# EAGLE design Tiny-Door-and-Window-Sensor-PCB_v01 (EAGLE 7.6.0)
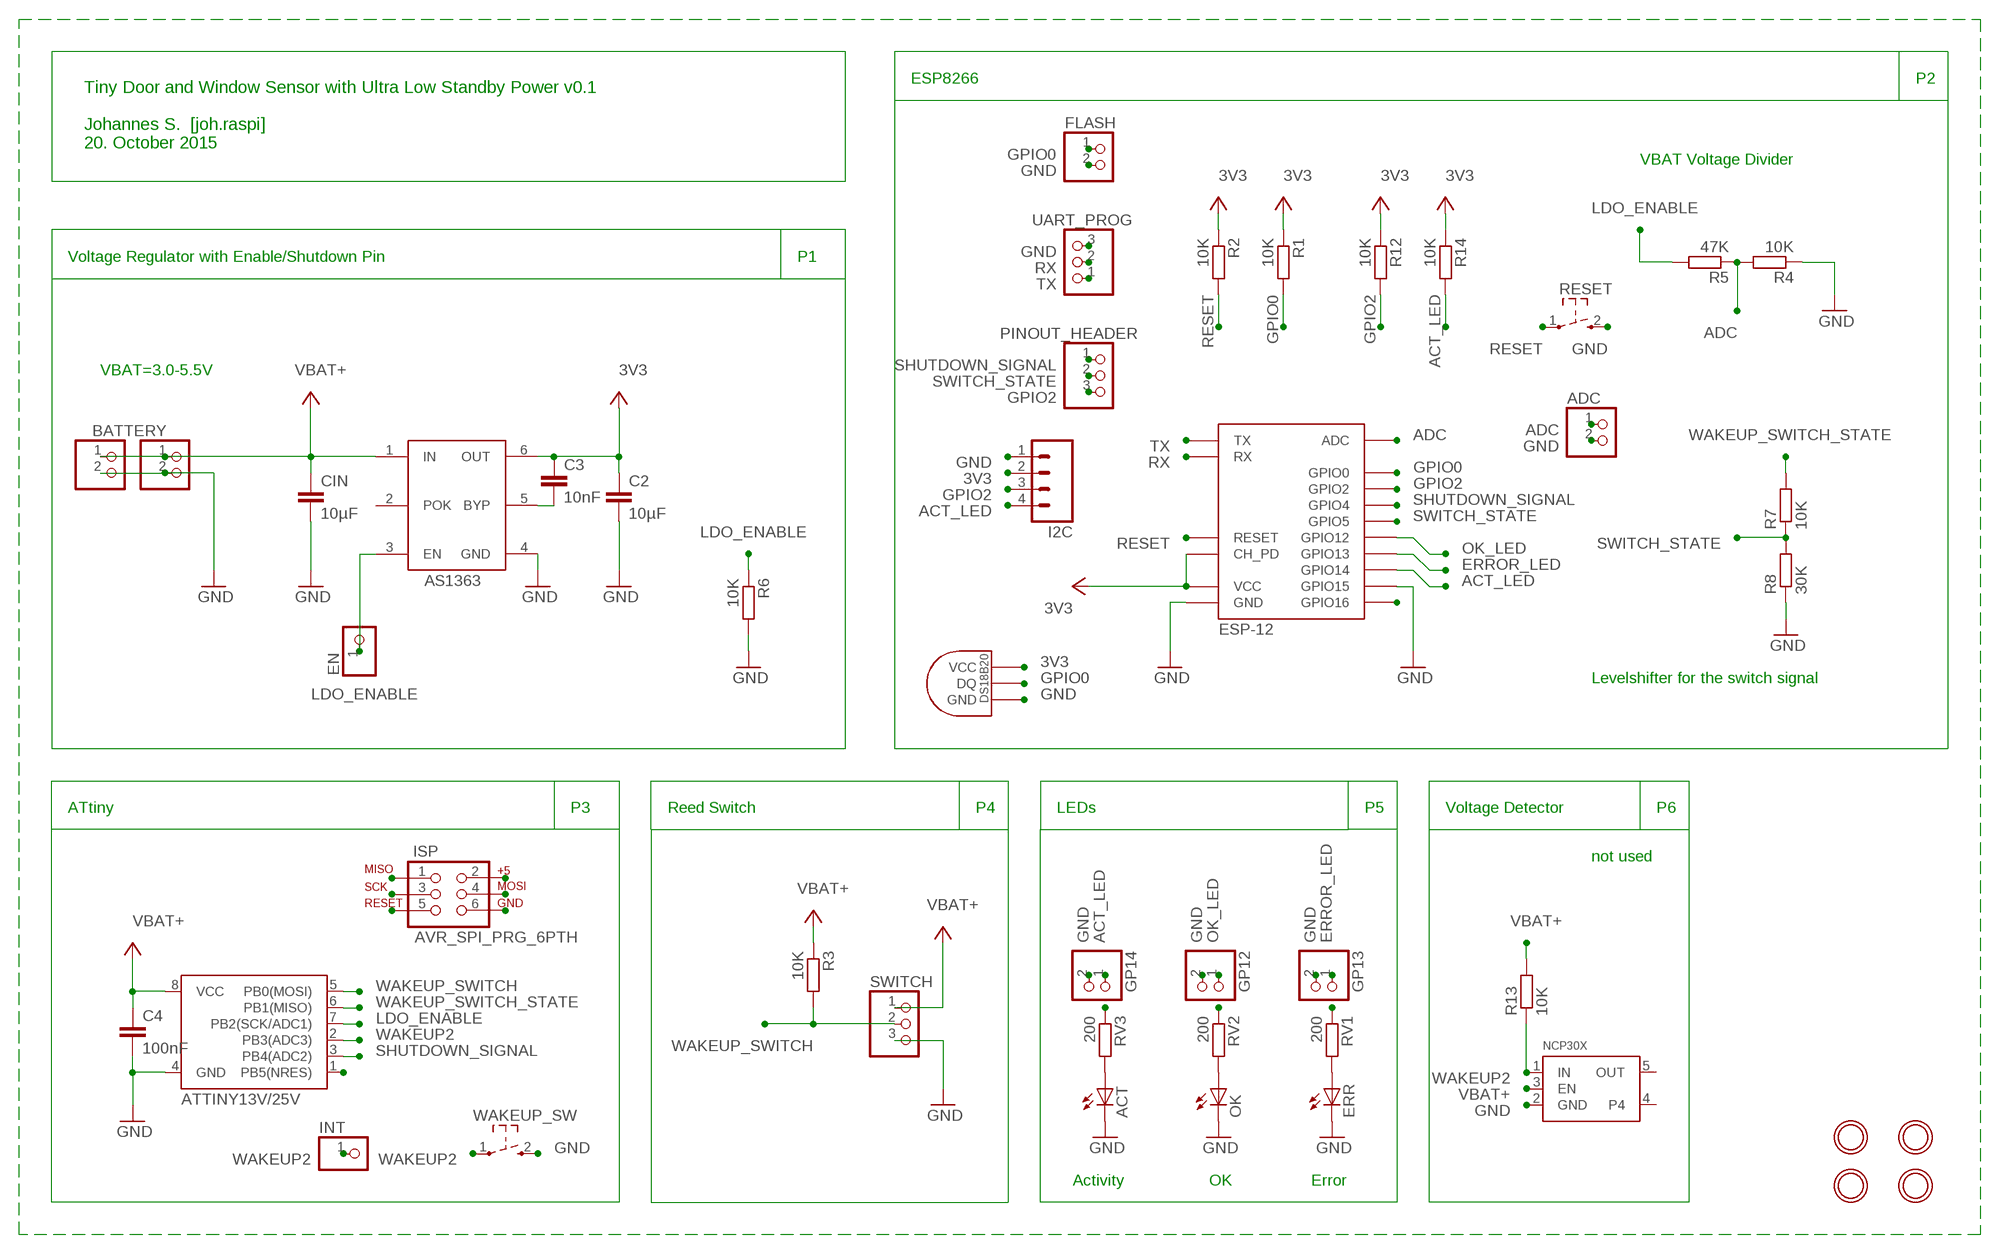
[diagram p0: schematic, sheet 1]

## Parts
ACT  LEDSML0805  [SML0805]
ADC  HEADER-1X2ROUND  [1X02_ROUND]
BATTERY  HEADER-1X2  [1X02_OVAL]
C2  10µF  C-EUC0805  [C0805]
C3  10nF  C-EUC0805  [C0805]
C4  100nF  C-EUC0805  [C0805]
CHARGE  HEADER-1X2  [1X02_OVAL]
CIN  10µF  C-EUC0805  [C0805]
EN  PINHD-1X1  [1X01]
ERR  LEDSML0805  [SML0805]
FLASH  HEADER-1X2ROUND  [1X02_ROUND]
GP12  HEADER-1X2ROUND  [1X02_ROUND]
GP13  HEADER-1X2ROUND  [1X02_ROUND]
GP14  HEADER-1X2ROUND  [1X02_ROUND]
I2C  M04PTH  [1X04]
IC1  AS1363  [SOT23-6]
INT  PINHD-1X1  [1X01]
ISP  AVR_SPI_PRG_6PTH  [2X3]
NCP30X  VREG_SOT23-5  [SOT23-5]
OK  LEDSML0805  [SML0805]
PINOUT_HEADER  PINHD-1X3  [1X03]
R1  10K  R-EU_R0805  [R0805]
R2  10K  R-EU_R0805  [R0805]
R3  10K  R-EU_R0805  [R0805]
R4  10K  R-EU_R0805  [R0805]
R5  47K  R-EU_R0805  [R0805]
R6  10K  R-EU_R0805  [R0805]
R7  10K  R-EU_R0805  [R0805]
R8  30K  R-EU_R0805  [R0805]
R12  10K  R-EU_R0805  [R0805]
R13  10K  R-EU_R0805  [R0805]
R14  10K  R-EU_R0805  [R0805]
RESET  SW_TACT_2P-3X6  [SW_TACT_3X6]
RV1  200  R-EU_R0805  [R0805]
RV2  200  R-EU_R0805  [R0805]
RV3  200  R-EU_R0805  [R0805]
SWITCH  PINHD-1X3  [1X03]
U$1  DS1820TO92  [DS1820]
U$2  ATTINY13V/25V  ATTINY13SOIC  [SO08]
U$3  ESP-12  [ESP-12]
U$4  MOUNTINGHOLE2.5_THICK  [MOUNTINGHOLE_2.5_PLATED_THICK]
U$5  MOUNTINGHOLE2.5_THICK  [MOUNTINGHOLE_2.5_PLATED_THICK]
U$6  MOUNTINGHOLE2.5_THICK  [MOUNTINGHOLE_2.5_PLATED_THICK]
U$7  MOUNTINGHOLE2.5_THICK  [MOUNTINGHOLE_2.5_PLATED_THICK]
UART_PROG  PINHD-1X3  [1X03]
WAKEUP_SW  SW_TACT_2P-3X6  [SW_TACT_3X6]

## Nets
3V3: C2.1 C3.1 I2C.2 IC1.6(OUT) R1.1 R2.1 R12.1 R14.1 U$1.VDD(VCC) U$3.CH_PD U$3.VCC ; supply symbol labelled VCC
ACT_LED: GP14.1 I2C.4 R14.2 RV3.1 U$3.GPIO14
ADC: ADC.1 R4.2 R5.1 U$3.ADC
AT_RESET: ISP.5 U$2.1(PB5(NRES))
ERROR_LED: GP13.1 RV1.1 U$3.GPIO13
GND: ACT.C ADC.2 BATTERY.2 C2.2 C4.2 CHARGE.2 CIN.2 ERR.C FLASH.2 GP12.2 GP13.2 GP14.2 I2C.1 IC1.4(GND) ISP.6 NCP30X.2(GND) OK.C R4.1 R6.2 R8.1 RESET.2 SWITCH.3 U$1.GND U$2.4(GND) U$3.GND U$3.GPIO15 UART_PROG.3 WAKEUP_SW.2
GPIO0: FLASH.1 R1.2 U$1.DQ U$3.GPIO0
GPIO2: I2C.3 PINOUT_HEADER.3 R12.2 U$3.GPIO2
LDO_ENABLE: EN.1 IC1.3(EN) ISP.3 R5.2 R6.1 U$2.7(PB2(SCK/ADC1))
N$4: C3.2 IC1.5(BYP)
N$8: ACT.A RV3.2
N$10: OK.A RV2.2
N$11: ERR.A RV1.2
N$15: U$3.GPIO16
OK_LED: GP12.1 RV2.1 U$3.GPIO12
RESET: R2.2 RESET.1 U$3.RESET
RX: U$3.RX UART_PROG.2
SHUTDOWN_SIGNAL: PINOUT_HEADER.1 U$2.3(PB4(ADC2)) U$3.GPIO4
SWITCH_STATE: PINOUT_HEADER.2 R7.1 R8.2 U$3.GPIO5
TX: U$3.TX UART_PROG.1
VBAT+: BATTERY.1 C4.1 CHARGE.1 CIN.1 IC1.1(IN) ISP.2 NCP30X.3(EN) R3.1 R13.2 SWITCH.1 U$2.8(VCC) ; supply symbol labelled VCC
WAKEUP2: INT.1 NCP30X.1(IN) R13.1 U$2.2(PB3(ADC3)) WAKEUP_SW.1
WAKEUP_SWITCH: ISP.4 R3.2 SWITCH.2 U$2.5(PB0(MOSI))
WAKEUP_SWITCH_STATE: ISP.1 R7.2 U$2.6(PB1(MISO))
Unconnected: IC1.2(POK) NCP30X.4 NCP30X.5(OUT)

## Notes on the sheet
- ESP8266 | P2
- Tiny Door and Window Sensor with Ultra Low Standby Power v0.1
  
  Johannes S.  [joh.raspi]
  20. October 2015
- VBAT Voltage Divider
- Voltage Regulator with Enable/Shutdown Pin | P1
- VBAT=3.0-5.5V
- Levelshifter for the switch signal
- ATtiny | P3 | Reed Switch | P4 | LEDs | P5 | Voltage Detector | P6
- not used
- Activity | OK | Error

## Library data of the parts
ACT ERR OK = led:LED: LED
ADC BATTERY CHARGE FLASH GP12-GP14 = microbuilder:HEADER-1X2: PIN HEADER
C2-C4 CIN = resistor:C-EU: CAPACITOR, European symbol
EN INT = pinhead:PINHD-1X1: PIN HEADER
I2C = SparkFun:M04: Header 4 Standard 4-pin 0.1" header. Use with straight break away headers (SKU : PRT-00116), right angle break away headers (PRT-00553), swiss pins (PRT-00743), machine pins (PRT-00117), and female headers (PRT-00115). Molex polarized connector foot print use with SKU : PRT-08231 with associated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
IC1 = joh_as1363:AS1363: 500mA ultra-low-dropout linear regulator 1.2V-5V 40µA quiescen current Source: http://ams.com/eng/content/download/12507/219217/12422
ISP = SparkFun:AVR_SPI_PRG_6: AVR ISP 6 Pin This is the reduced ISP connector for AVR programming. Common on Arduino. This footprint will take up less PCB space and can be used with a 10-pin to 6-pin adapter such as SKU: BOB-08508
NCP30X = microbuilder:VREG_SOT23-5: SOT23-5 Fixed Voltage Regulators To better organise some of the SOT23-5 fixed voltage regulators in this library, this new part was created. Part Current Out V Out V In V Dropout Digikey Part No. ADP121 150mA 3.3V 3.4-5.5V 0.09V @ 150mA ADP121-AUJZ33R7CT-ND ADP121 150mA 3.0V 3.1-5.5V 0.09V @ 150mA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
PINOUT_HEADER SWITCH UART_PROG = pinhead:PINHD-1X3: PIN HEADER
R1-R8 R12-R14 RV1-RV3 = resistor:R-EU_: RESISTOR, European symbol
RESET WAKEUP_SW = dp-devices:SW_TACT_2P
U$1 = Ava:DS1820: DS18B20 Programmable Resolution 1-Wire Digital Thermometer Description The DS18B20 digital thermometer provides 9-bit to 12-bit Celsius temperature measurements and has an alarm function with nonvolatile user-programmable upper and lower trigger points. The DS18B20 communicates over a 1-Wire® bus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
U$2 = SparkFun:ATTINY13
U$3 = johs_esp8266_lib_frank_esp12e_mod:ESP-12: ESP8266 Wifi Module ESP-12; DIMENSIONS: 24.0 x 16.0 mm; PINS: 16; PITCH: 0.078" / 2 mm
U$4-U$7 = microbuilder:MOUNTINGHOLE: Mounting Hole

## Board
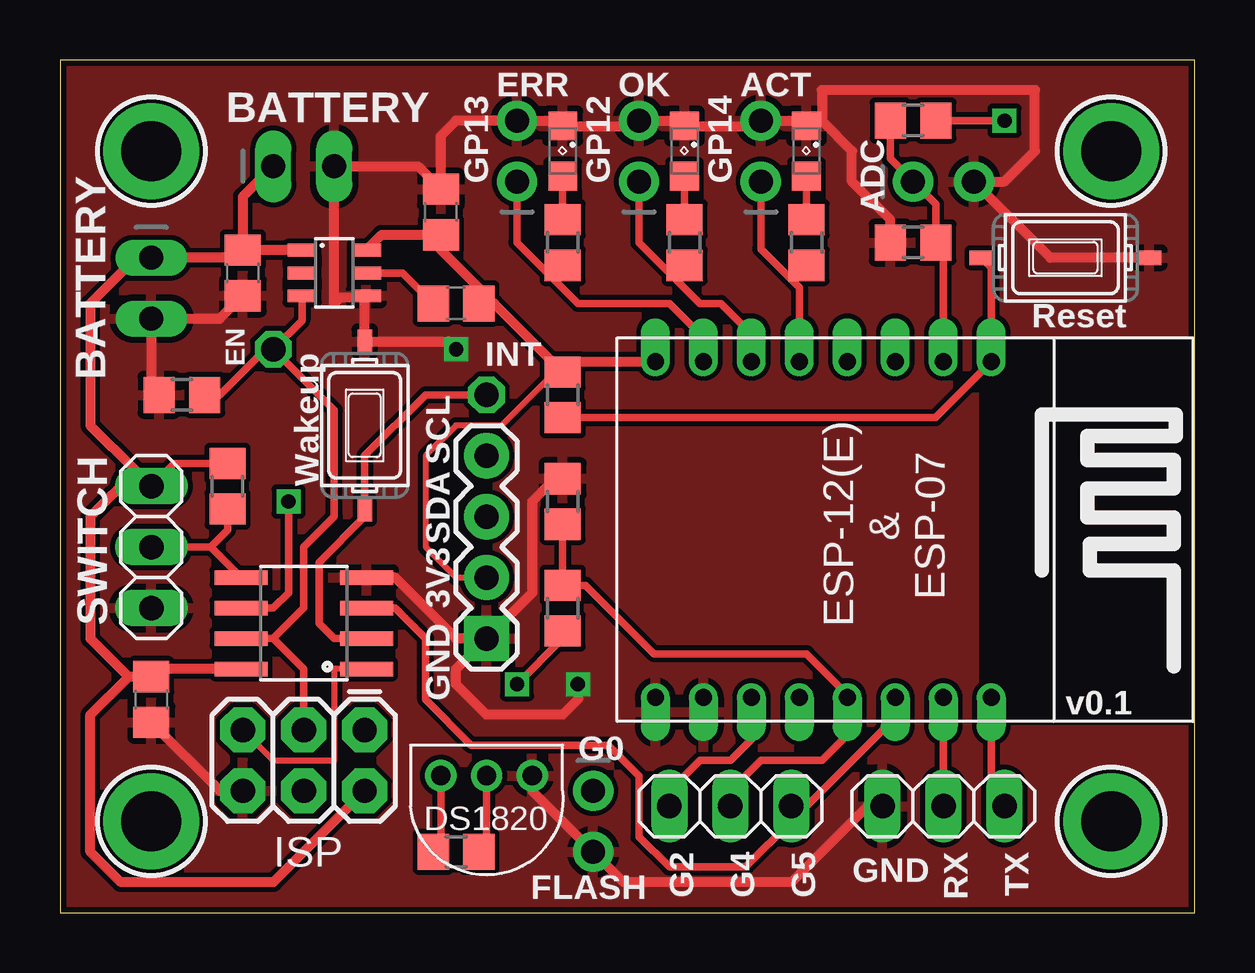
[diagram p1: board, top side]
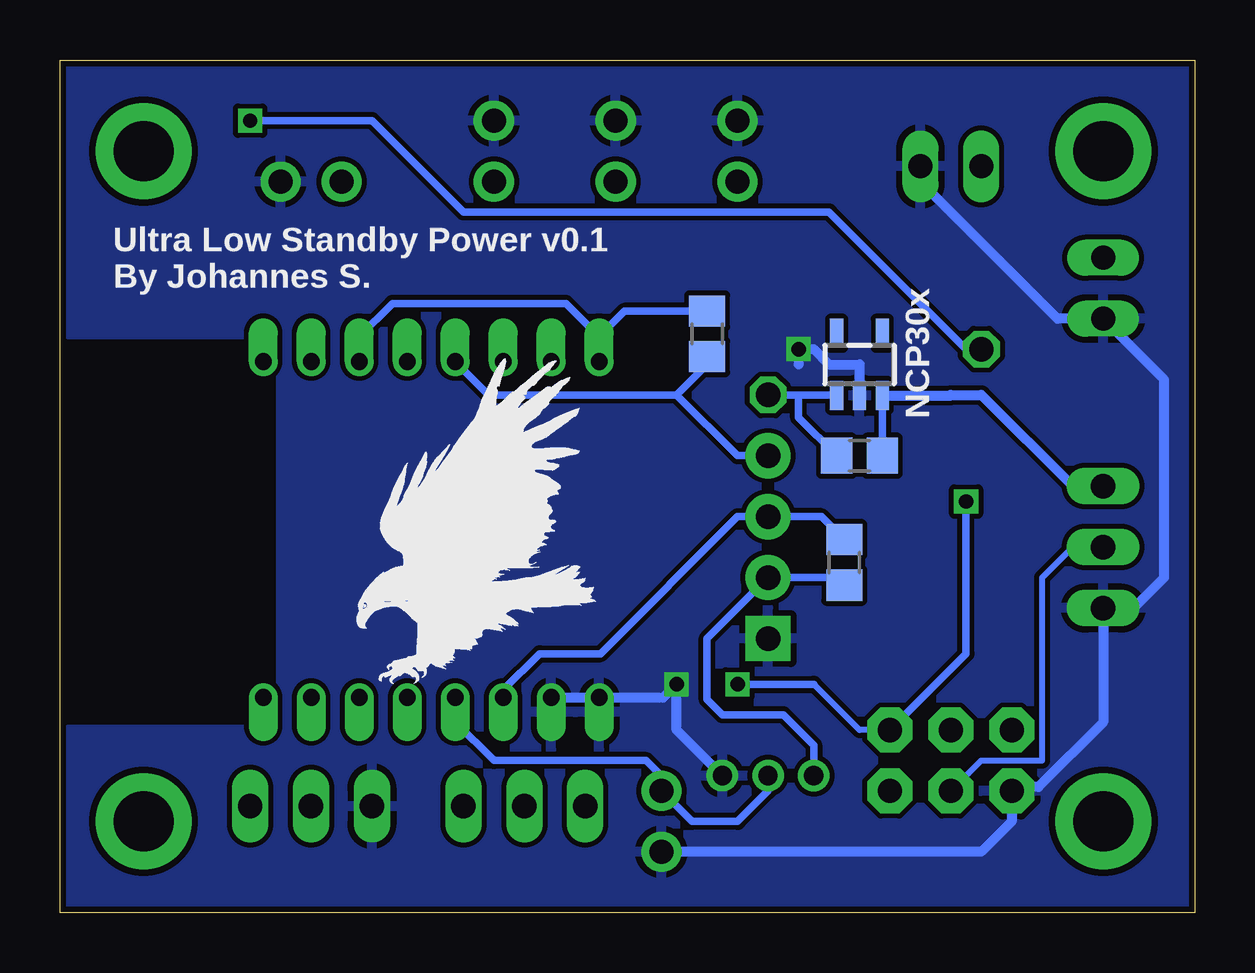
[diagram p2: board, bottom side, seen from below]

Size 47.3 x 35.55 mm. Coordinates in mm from the lower left corner, seen from the top.
Outline: 0,0 47.3,0 47.3,35.55 0,35.55 0,0
Copper layers (1*16): Top 0.035mm / dielectric 1.5mm / Bottom 0.035mm
Design rules "adafruit": minimum track width 10mil, minimum drill 15.5mil, track to track 8mil, track to pad 8mil, pad to pad 8mil, via to via 8mil, smd to smd 8mil, copper to edge 10mil, drill to drill 8mil, minimum pad ring 10mil, minimum via ring 8mil, stop-mask expansion 2mil, vias tented up to drill 20mil, thermal gap 10mil

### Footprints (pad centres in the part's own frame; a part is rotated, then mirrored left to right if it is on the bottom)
SML0805 = smd 1.2 x 1.2: A 1.05,0; C -1.05,0
1X02_ROUND = drill 1 pad 1.676: 1 -1.27,0; 2 1.27,0
1X02_OVAL = drill 1 long: 1 -1.27,0; 2 1.27,0
C0805 = smd 1.3 x 1.5: 1 -0.95,0; 2 0.95,0
1X01 = drill 1.016 octagon: 1 0,0
1X04 = drill 1.016 pad 1.88 square: 1 0,0 | drill 1.016 pad 1.88: 2 2.54,0; 3 5.08,0; 4 7.62,0
SOT23-6 = smd 0.533 x 1.219: 1 -0.95,-1.341; 2 0,-1.341; 3 0.95,-1.341; 4 0.95,1.341; 5 0,1.341; 6 -0.95,1.341
2X3 = drill 1.016 pad 1.88 octagon: 1 0,0; 2 0,2.54; 3 2.54,0; 4 2.54,2.54; 5 5.08,0; 6 5.08,2.54
SOT23-5 = smd 0.55 x 1.2: 1 -0.95,-1.3; 2 0,-1.3; 3 0.95,-1.3; 4 0.95,1.3; 5 -0.95,1.3
1X03 = drill 1.016 long: 1 -2.54,0; 2 0,0; 3 2.54,0
R0805 = smd 1.3 x 1.5: 1 -0.95,0; 2 0.95,0
SW_TACT_3X6 = smd 1 x 0.6: 1 -3.5,0; 2 3.5,0
DS1820 = drill 0.8: DQ 2.54,-1.27; GND 0.635,-1.27; VDD 4.445,-1.27
SO08 = smd 0.61 x 2.21: 1 -1.905,-2.616; 2 -0.635,-2.616; 3 0.635,-2.616; 4 1.905,-2.616; 5 1.905,2.616; 6 0.635,2.616; 7 -0.635,2.616; 8 -1.905,2.616
ESP-12 = drill 0.7 offset: ADC -7.1,3.8; CH_PD -7.1,1.8; GND 6.9,-8.2; GPIO0 6.9,-2.2; GPIO2 6.9,-4.2; GPIO4 6.9,1.8; GPIO5 6.9,-0.2; GPIO12 -7.1,-4.2; GPIO13 -7.1,-6.2; GPIO14 -7.1,-2.2; GPIO15 6.9,-6.2; GPIO16 -7.1,-0.2; RESET -7.1,5.8; RX 6.9,3.8; TX 6.9,5.8; VCC -7.1,-8.2
MOUNTINGHOLE_2.5_PLATED_THICK = drill 2.5 pad 4: P$1 0,0

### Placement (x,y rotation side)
ACT  31.11,31.75 270 top
ADC  36.83,30.48 0 top
BATTERY  10.16,31.11 0 top
C2  15.88,29.21 90 top
C3  16.51,25.4 180 top
C4  3.81,8.89 270 top
CHARGE  3.81,26.04 270 top
CIN  7.62,26.67 270 top
EN  8.89,23.5 0 top
ERR  20.95,31.75 270 top
FLASH  22.23,3.81 270 top
GP12  24.13,31.75 90 top
GP13  19.05,31.75 90 top
GP14  29.21,31.75 90 top
I2C  17.78,11.43 90 top
IC1  11.43,26.67 270 top
INT  17.78,21.59 0 top
ISP  12.7,7.62 180 top
NCP30X  13.97,22.86 0 bottom
OK  26.04,31.75 270 top
PINOUT_HEADER  27.94,4.45 180 top
R1  16.51,2.54 0 top
R2  20.95,21.59 270 top
R3  6.99,17.78 270 top
R4  35.56,27.94 0 top
R5  35.56,33.02 0 top
R6  5.08,21.59 180 top
R7  20.95,12.7 270 top
R8  20.95,17.14 270 top
R12  14.61,14.61 90 bottom
R13  13.97,19.05 0 bottom
R14  20.32,24.13 270 bottom
RESET  41.91,27.3 0 top
RV1  20.95,27.94 90 top
RV2  26.04,27.94 90 top
RV3  31.11,27.94 90 top
SWITCH  3.81,15.24 270 top
U$1  20.32,4.45 180 top
U$2  10.16,12.06 90 top
U$3  33.02,15.88 270 top
U$4  43.81,31.75 0 top
U$5  3.81,3.81 0 top
U$6  43.81,3.81 0 top
U$7  3.81,31.75 0 top
U$9  [EAGLE-PLC-10MM]  34.92,9.53 0 bottom
UART_PROG  36.83,4.45 180 top
WAKEUP_SW  12.7,20.32 90 top

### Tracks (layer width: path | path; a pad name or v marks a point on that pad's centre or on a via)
3V3
  Top 0.254: 20.64,22.54 18.41,20.32 16.51,20.32 15.24,19.05 15.24,15.24 16.51,13.97 I2C.2
  Top 0.305: U$1.VDD 15.88,2.85 R1.1 | R2.1 20.64,22.54
  Top 0.406: IC1.6 13.41,28.26 C2.1 15.88,27.62 17.46,26.04 C3.1 18.09,25.4 R2.1 21.39,22.98 U$3.VCC
  Bottom 0.305: U$3.VCC 24.82,24.02 | 24.82,24.02 26.2,25.4 33.44,25.4 34.82,24.02 U$3.CH_PD | U$1.VDD 15.88,6.99 17.14,8.26 19.68,8.26 20.32,8.89 20.32,11.43 I2C.2 14.92,13.97 R12.1 | R14.1 23.75,25.08 24.82,24.02
ACT_LED
  Top 0.305: U$3.GPIO14 30.82,26.06 30.34,26.54 | GP14.1 29.21,27.67 30.34,26.54 | RV3.1 30.8,26.99 30.34,26.54
  Bottom 0.305: 21.59,21.59 19.05,19.05 I2C.4 | 21.59,21.59 29.43,21.59 U$3.GPIO14 | R14.2 20.32,22.86 21.59,21.59
ADC
  Top 0.305: U$3.ADC 36.82,27.63 R4.2 36.51,29.53 ADC.1 34.61,31.43 R5.1
AT_RESET
  Top 0.254: ISP.5 8.89,6.35 11.43,6.35 11.43,10.16 U$2.1
ERROR_LED
  Top 0.305: U$3.GPIO13 26.82,23.98 25.4,25.4 21.59,25.4 20.32,26.67 | GP13.1 19.05,27.94 20.32,26.67 | RV1.1 20.64,26.99 20.32,26.67
GND  (via drill 0.6)
  Top 0.406: UART_PROG.3 33.66,4.45 30.48,1.27 23.5,1.27 FLASH.2 19.68,5.08 U$1.GND | R4.1 34.61,28.89 33.02,30.48 33.02,31.75 31.75,33.02 | 31.75,33.02 31.34,33.02 ACT.C 30.89,33.02 GP14.2 28.99,32.8 OK.C 25.82,33.02 GP12.2 23.91,32.8 ERR.C 20.73,33.02 GP13.2 16.51,33.02 15.88,32.38 C2.2 14.92,31.11 BATTERY.2 11.43,25.4 11.68,25.65 12.7,25.65 | RESET.2 41.27,27.3 ADC.2 39.37,30.48 40.64,31.75 40.64,34.29 31.75,34.29 31.75,33.02 | R6.2 3.81,21.91 CHARGE.2 6.67,24.77 CIN.2 7.62,25.4 | 12.7,25.65 WAKEUP_SW.2 16.18,23.82 v16.51,23.5 | 12.7,25.65 IC1.4 | I2C.1 16.51,11.43 13.97,13.97 U$2.4 | R8.1 20.64,18.09 19.68,17.14 19.68,13.34 I2C.1 | ISP.6 6.67,5.08 C4.2 | v21.59,9.53 21.59,8.89 20.95,8.26 17.78,8.26 16.51,9.53 16.51,10.16 I2C.1
  Bottom 0.305: 22.31,8.97 22.14,8.97
  Bottom 0.406: U$3.GPIO15 U$3.GND 22.31,8.97 | 22.14,8.97 v21.59,9.53 21.59,7.62 U$1.GND | NCP30X.2 13.97,22.86 15.24,22.86 15.88,23.5 v16.51,23.5 16.51,22.86 | 11.43,30.48 5.71,24.77 CHARGE.2 1.27,22.23 1.27,13.97 2.54,12.7 SWITCH.3 C4.2 6.51,5.24 7.46,5.24 ISP.6 7.62,3.81 8.89,2.54 FLASH.2
  pour Top: 0,35.56 46.99,35.56 46.99,24.13 38.1,24.13 38.1,7.62 46.99,7.62 46.99,0 0,0
  pour Bottom: 0,35.56 46.99,35.56 46.99,24.13 38.1,24.13 38.1,7.62 46.99,7.62 46.99,0 0,0
GPIO0
  Top 0.305: U$1.DQ 17.78,2.86 R1.2
  Bottom 0.305: U$3.GPIO0 30.82,7.96 29.21,6.35 22.86,6.35 22.23,5.71 FLASH.1 20.95,3.81 19.05,3.81 17.78,5.08 U$1.DQ
GPIO2
  Top 0.305: PINOUT_HEADER.3 25.4,5.08 26.67,6.35 27.94,6.35 28.82,7.23 U$3.GPIO2
  Bottom 0.305: U$3.GPIO2 28.82,9.28 27.3,10.79 24.77,10.79 19.05,16.51 I2C.3 15.56,16.51 R12.2
LDO_ENABLE  (via drill 0.6)
  Top 0.305: v39.37,33.02 R5.2 | U$2.7 8.89,11.43 | 8.89,11.43 10.16,12.7 10.16,15.24 11.43,16.51 11.43,20.95 EN.1 | R6.1 6.66,21.59 6.67,21.59 8.57,23.5 EN.1 | ISP.3 10.16,10.16 8.89,11.43 | IC1.3 10.09,24.7 EN.1
  Bottom 0.305: v39.37,33.02 34.29,33.02 30.48,29.21 15.24,29.21 9.53,23.5 EN.1
N$4
  Top 0.305: IC1.5 14.29,26.67 C3.2
N$8
  Top 0.305: ACT.A RV3.2
N$10
  Top 0.305: OK.A RV2.2
N$11
  Top 0.305: ERR.A RV1.2
OK_LED
  Top 0.305: U$3.GPIO12 28.82,24.13 27.55,25.4 26.67,25.4 25.4,26.67 | GP12.1 24.13,27.94 25.4,26.67 | RV2.1 26.04,26.91 25.64,26.91 25.4,26.67
RESET
  Top 0.305: RESET.1 38.82,26.89 U$3.RESET 36.48,20.64 R2.2
RX
  Top 0.305: UART_PROG.2 U$3.RX
SHUTDOWN_SIGNAL
  Top 0.305: U$3.GPIO4 34.82,8.15 31.11,4.45 PINOUT_HEADER.1 30.48,3.81 28.57,1.91 25.4,1.91 24.13,3.17 24.13,5.71 22.86,6.99 17.14,6.99 15.24,8.89 15.24,11.43 13.97,12.7 U$2.3
SWITCH_STATE
  Top 0.305: PINOUT_HEADER.2 27.94,5.08 29.21,6.35 31.75,6.35 32.82,7.42 U$3.GPIO5 32.82,9.09 31.11,10.79 24.77,10.79 21.91,13.65 R7.1 R8.2
TX
  Top 0.305: U$3.TX 38.82,5 UART_PROG.1
VBAT+
  Top 0.305: CIN.1 7.62,27.94 | R3.1 4.76,18.73 SWITCH.1
  Top 0.406: IC1.1 CIN.1 7.3,27.3 CHARGE.1 3.17,27.3 1.27,25.4 1.27,20.32 3.17,18.41 | BATTERY.1 7.62,29.84 7.62,27.94 | SWITCH.1 3.17,18.41 | 3.17,18.41 1.27,16.51 1.27,11.43 2.86,9.84 | U$2.8 4.13,10.16 C4.1 2.86,9.84 | ISP.2 8.89,1.27 2.54,1.27 1.27,2.54 1.27,8.25 2.86,9.84
  Bottom 0.305: NCP30X.3 R13.2
  Bottom 0.406: NCP30X.3 10.19,21.56 10.16,21.59 8.89,21.59 5.08,17.78 SWITCH.1
WAKEUP2
  Top 0.305: INT.1 15.24,21.59 12.7,19.05 WAKEUP_SW.1 12.7,16.51 10.79,14.61 10.79,12.06 11.43,11.43 U$2.2
  Bottom 0.305: 14.95,21.59 16.51,21.59 | 16.51,21.59 INT.1 | R13.1 16.51,20.64 16.51,21.59
  Bottom 0.406: NCP30X.1 14.95,21.59
WAKEUP_SWITCH
  Top 0.305: 2.54,15.24 SWITCH.2 6.27,15.24 | 6.27,15.24 U$2.5 | R3.2 6.99,15.95 6.27,15.24
  Bottom 0.254: ISP.4 8.89,6.35 6.35,6.35 6.35,13.97 5.08,15.24 SWITCH.2
WAKEUP_SWITCH_STATE  (via drill 0.6)
  Top 0.305: U$2.6 8.89,12.7 9.53,13.34 v9.53,17.14 | R7.2 20.95,11.43 v19.05,9.53
  Bottom 0.254: ISP.1 13.97,7.62 15.88,9.53
  Bottom 0.305: v19.05,9.53 15.88,9.53 | ISP.1 9.53,10.79 v9.53,17.14

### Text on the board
tPlace: Reset | BATTERY | SCL | Wakeup | SDA | 3V3 | GND | v0.1 | G0 | G2 | G4 | G5 | RX | TX | GND
bPlace: NCP30x | Ultra Low Standby Power v0.1 / By Johannes S.

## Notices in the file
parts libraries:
SparkFun: Licensing: CC v3.0 Share-Alike You are welcome to use this library for commercial purposes.
microbuilder: This work is placed in the public domain, and may be freely used for commercial and non-commercial work with the following conditions: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
